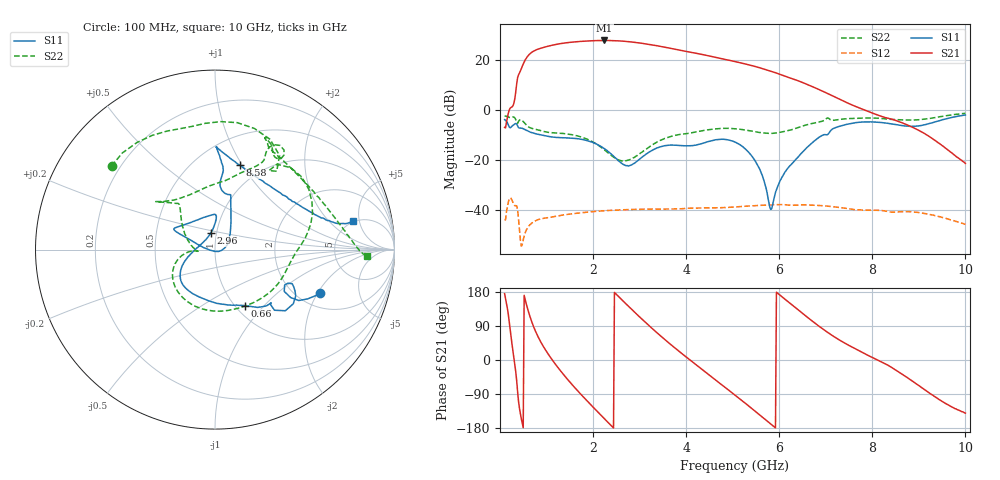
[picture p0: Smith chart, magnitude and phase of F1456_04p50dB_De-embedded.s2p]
! Integrated Device Technology
! Corporate Headquarters
! 6024 Silver Creek Valley Road
! San Jose, CA 95138  USA
! Phone:  1-408-284-8200
! Toll Free:  1-800-223-1366
! Webpage:  http://www.idt.com/
! Timing and RF Division
! 515 Groton Road, Suite 102
! Westford, MA 01886-6024
! Device:  F1456
! Description: 6-bit 0.5 dB Transmit Variable Gain Amplifier
! Frequency:  2100.0 -  2950.00 MHz
! Package:  6x6 mm Thin QFN Plastic Package: 28 pin
! State:  9
! Atten State:  4.5 dB
! Voltage:  +5.00 Volts
! Current:  215.459 mA
! Data:  The device was measured on a the F1455 evaluation board which has
!  individual transmission lines to the RF pins.  Data was collected
!  using a calibrated network analyzer.  The evaluation board was
!  de-embedded using a TRL calibration technique.
!  The reference plane is the edge of the package pin.
!  Pin  1 = CSb
!  Pin  2 = DATA
!  Pin  3 = CLK
!  Pin  4 = RSET
!  Pin  5 = GND
!  Pin  6 = RFIN  = Port 1
!  Pin  7 = GND
!  Pin  8 = NC
!  Pin  9 = NC
!  Pin 10 = NC
!  Pin 11 = NC
!  Pin 12 = NC
!  Pin 13 = NC
!  Pin 14 = /STBY
!  Pin 15 = GND
!  Pin 16 = RFOUT  = Port 2
!  Pin 17 = GND
!  Pin 18 = NC
!  Pin 19 = NC
!  Pin 20 = NC
!  Pin 21 = GND
!  Pin 22 = NC
!  Pin 23 = GND
!  Pin 24 = NC
!  Pin 25 = NC
!  Pin 26 = NC
!  Pin 27 = GND
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# GHz S dB R 50
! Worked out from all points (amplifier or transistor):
!   496 points, 100 MHz to 10 GHz, reference 50 ohm
!   highest |S21| = 27.7 dB at 2.24 GHz (marker M1)
!   |S21| within 3 dB of that: 896 MHz to 3.624 GHz (2.728 GHz wide, 121 % of centre)
!   unconditionally stable (mu >= 1): start of sweep to end of sweep
!   at 1.74 GHz: K = 2.28, MAG = 27.9 dB, |S12| = -41.2 dB
!   at 5.06 GHz: K = 3.93, MAG = 20.2 dB, |S12| = -38.9 dB
!   at 10 GHz: K = 129.16, MAG = -12.0 dB, |S12| = -45.8 dB
!   S11 on the Smith chart (normalised r, x): 100 MHz: 2.57, -2.09; 660 MHz: 1.10, -0.79; 2.96 GHz: 0.94, +0.18; 8.58 GHz: 0.79, +0.98; 10 GHz: 4.90, +4.00
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0.1  -3.99 -22.8  -7.09 174.9  -43.89 43.0  -2.61 141.1
0.34  -5.51 -34.6  7.20 -31.6  -38.38 -145.1  -3.94 55.5
0.42  -7.32 -43.5  14.71 -128.4  -48.25 140.0  -4.13 47.2
0.54  -7.95 -53.6  19.82 160.5  -49.38 -169.3  -5.56 10.8
0.66  -9.04 -61.9  22.63 109.0  -45.73 156.9  -7.31 -7.6
0.84  -9.94 -75.8  24.37 56.2  -43.86 114.4  -8.19 -35.8
1.16  -10.99 -102.7  25.94 -6.0  -42.78 70.1  -9.25 -83.4
1.48  -11.32 -123.9  26.89 -55.1  -41.79 42.2  -9.80 -122.3
1.76  -11.89 -138.8  27.35 -93.4  -41.17 22.8  -10.98 -146.8
1.98  -12.98 -148.7  27.58 -121.7  -40.80 9.2  -12.73 -161.6
2.24  -15.53 -162.0  27.70 -154.4  -40.41 -5.7  -15.97 -173.8
2.56  -20.64 169.5  27.52 166.0  -40.09 -23.2  -20.19 -174.9
2.96  -20.39 104.1  26.80 118.3  -39.83 -43.8  -18.12 174.1
3.4  -15.15 87.7  25.49 69.0  -39.74 -65.0  -12.73 142.2
4.04  -14.44 111.3  23.17 4.2  -39.41 -92.3  -9.49 129.9
4.54  -12.42 147.6  21.32 -44.1  -39.29 -114.8  -7.86 139.1
5.06  -13.01 155.8  19.21 -93.6  -38.89 -136.7  -7.62 140.0
5.72  -31.56 -172.5  15.99 -159.0  -38.17 -171.3  -9.40 118.5
6.7  -13.36 65.7  9.33 103.7  -38.14 128.7  -5.53 63.0
8.36  -5.52 83.1  -3.50 -15.4  -40.88 54.6  -3.81 62.4
8.58  -6.19 73.7  -4.83 -32.8  -40.85 49.3  -4.02 56.6
10  -2.11 11.6  -21.53 -140.2  -45.83 -27.6  -1.46 -2.5
